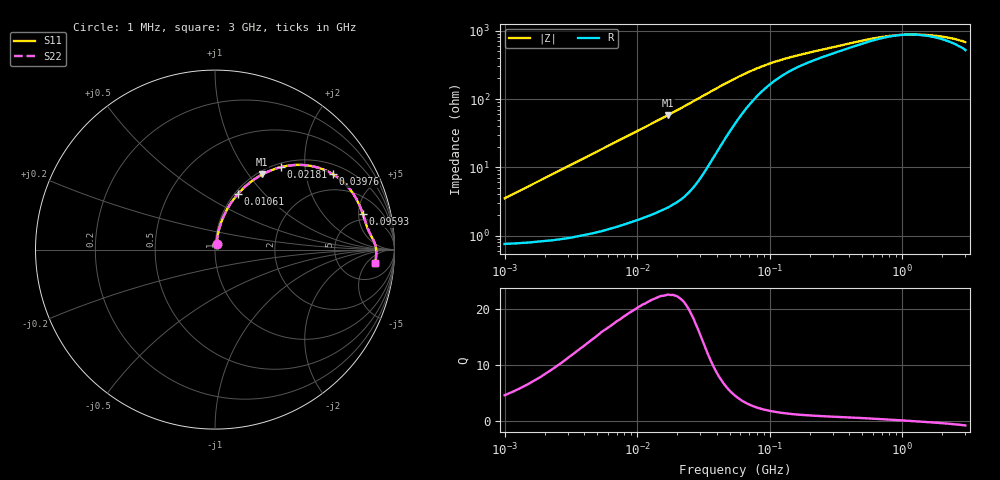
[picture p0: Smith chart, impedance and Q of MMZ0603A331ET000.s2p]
! S-Parameter Data Generated by TDK Corporation
! Copyright(C) 2025 TDK Corporation.
! All Rights Reserved.
! TDK P/N: MMZ0603A331ET000 (Chip Bead)
! Property: |Z|=330ohm at 100MHz
! Size(LxWxT): 0.6x0.3x0.3mm
! Model Type: s2p (Touchstone File Format Version 1.0)
! Frequency: DC=Yes Start=1MHz Stop=3000MHz 202points Log-sweep
! Model Generated on Feb. 6, 2025
! Terms and conditions regarding TDK Simulation Models:
! 1)This simulation model is being provided solely for informational
!  purposes. Please refer to the specifications of the products in
!  terms of detailed characteristics of such products.
! 2)In no event shall TDK Corporation of any of its subsidiaries be
!  liable for any loss or damage arising, directly or indirectly,
!  from any information contained in this simulation model, including,
!  but not limited to loss or damages arising from any inaccuracies,
!  omissions or errors in connection with such information.
! 3)Any and all copyrights on this simulation model are owned by
!  TDK Corporation.  Duplication or redistribution of this simulation
!  model without prior written permission from TDK Corporation
!  is prohibited.
! 4)This simulation model is subject to any modification or change
!  without any prior notice.
! 5)Neither TDK Corporation nor any of its subsidiaries shall make any
!  warranty, express or implied, including but not limited to the
!  correctness, implied warranties of merchantability and fitness for
!  a particular purpose with respect to this simulation models.
! 6)The use of this simulation model shall be deemed to have consented
!  to the terms and conditions hereof.
! Port Assignments:
!  1 ---@@@--- 2
! Applicable Conditions:
!  Temperature = 25 degC
!  DC Bias Current = 0 A
!  Small Signal Operation
# Hz S MA R 50
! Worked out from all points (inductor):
!   201 points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, 1 MHz to 3 GHz, reference 50 ohm
!   read as one part in series: L = 547 nH near 1.041 MHz
!   highest Q = 22.4 at 17.15 MHz (marker M1), where L = 540 nH
!   self-resonance near 1.096 GHz
!   S11 on the Smith chart (normalised r, x): 1 MHz: 1.02, +0.07; 10.61 MHz: 1.04, +0.72; 21.81 MHz: 1.07, +1.50; 39.76 MHz: 1.33, +2.85; 95.93 MHz: 4.04, +5.66; 3 GHz: 11, -9
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1000000  0.03491 75.7  0.9919 -2.0  0.9919 -2.0  0.03491 75.7
2139570  0.07301 79.3  0.989 -4.2  0.989 -4.2  0.07301 79.3
3900413  0.131 78.2  0.9815 -7.5  0.9815 -7.5  0.131 78.2
6831390  0.2233 73.9  0.9621 -12.9  0.9621 -12.9  0.2233 73.9
1.061086e7  0.3329 67.8  0.9269 -19.4  0.9269 -19.4  0.3329 67.8
1.461624e7  0.436 61.6  0.8805 -25.8  0.8805 -25.8  0.436 61.6
1.71545e7  0.4941 57.9  0.8477 -29.6  0.8477 -29.6  0.4941 57.9
2.181181e7  0.5864 51.5  0.7833 -35.9  0.7833 -35.9  0.5864 51.5
2.886629e7  0.6908 42.9  0.6819 -43.6  0.6819 -43.6  0.6908 42.9
3.387922e7  0.7407 37.7  0.6136 -47.6  0.6136 -47.6  0.7407 37.7
3.976269e7  0.7794 32.7  0.5432 -50.7  0.5432 -50.7  0.7794 32.7
5.477226e7  0.825 23.8  0.4133 -53.6  0.4133 -53.6  0.825 23.8
6.964249e7  0.8391 18.5  0.3362 -52.5  0.3362 -52.5  0.8391 18.5
9.593103e7  0.8476 13.4  0.264 -48.3  0.264 -48.3  0.8476 13.4
1.375402e8  0.8539 9.7  0.2134 -42.1  0.2134 -42.1  0.8539 9.7
2.136344e8  0.8634 6.7  0.1747 -35.4  0.1747 -35.4  0.8634 6.7
4.951867e8  0.8866 3.1  0.1242 -22.6  0.1242 -22.6  0.8866 3.1
8.005644e8  0.8952 1.2  0.1067 -10.2  0.1067 -10.2  0.8952 1.2
1.147801e9  0.8981 -0.2  0.1019 1.6  0.1019 1.6  0.8981 -0.2
1.581072e9  0.8986 -1.4  0.1042 12.5  0.1042 12.5  0.8986 -1.4
2.266846e9  0.8981 -3.1  0.1141 25.2  0.1141 25.2  0.8981 -3.1
3e9  0.8954 -4.9  0.1318 35.1  0.1318 35.1  0.8954 -4.9
